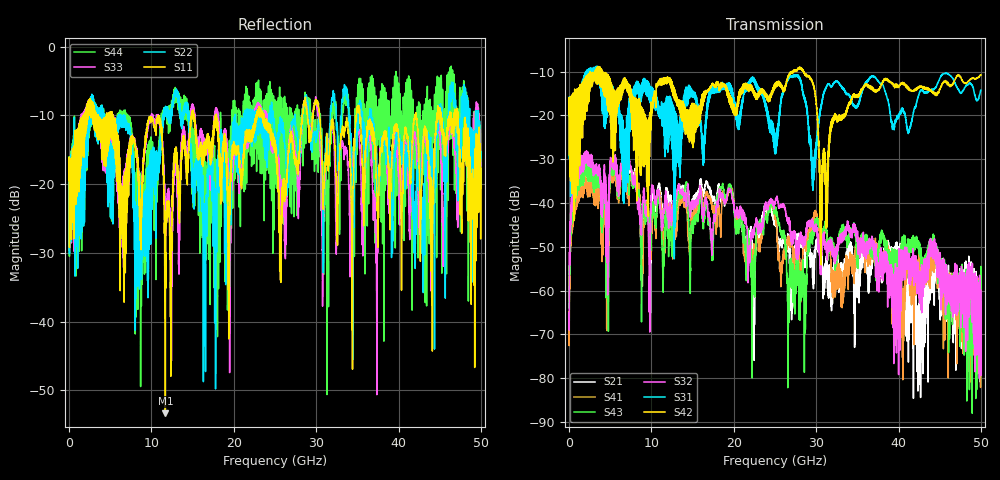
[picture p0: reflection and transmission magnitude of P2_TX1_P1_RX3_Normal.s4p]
!Keysight Technologies,N5225B,MY57041031,A.13.20.10
!Date: Friday, May 31, 2019 11:17:59
!Correction: S11(Full 4 Port(1,2,3,4))
!S12(Full 4 Port(1,2,3,4))
!S13(Full 4 Port(1,2,3,4))
!S14(Full 4 Port(1,2,3,4))
!S21(Full 4 Port(1,2,3,4))
!S22(Full 4 Port(1,2,3,4))
!S23(Full 4 Port(1,2,3,4))
!S24(Full 4 Port(1,2,3,4))
!S31(Full 4 Port(1,2,3,4))
!S32(Full 4 Port(1,2,3,4))
!S33(Full 4 Port(1,2,3,4))
!S34(Full 4 Port(1,2,3,4))
!S41(Full 4 Port(1,2,3,4))
!S42(Full 4 Port(1,2,3,4))
!S43(Full 4 Port(1,2,3,4))
!S44(Full 4 Port(1,2,3,4))
!S4P File: Measurements: <S11,S12,S13,S14>,
!<S21,S22,S23,S24>,
!<S31,S32,S33,S34>,
!<S41,S42,S43,S44>:
# Hz S  dB  R 50.0
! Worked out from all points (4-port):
!   5000 points, 10 MHz to 50 GHz, reference 50 ohm
!   strongest paths, dB at 10 MHz, 12.51 GHz, 25.01 GHz, 37.51 GHz, 50 GHz:
!     S42: -19.7, -14.1, -12.9, -14.2, -10.7
!     S31: -19.5, -17.3, -28.8, -12.1, -14.2
!     S32: -65.1, -42.4, -40.2, -56.7, -63.4
!     S43: -62.3, -46.9, -42.0, -50.8, -61.4
!     S41: -64.8, -44.4, -43.4, -51.4, -67.8
!     S21: -62.4, -42.2, -44.5, -52.7, -71.1
!   lowest |S11| = -53.4 dB at 11.69 GHz (marker M1), VSWR 1.00, Z = 49.8 - j0.101 ohm
!   |S11| at or under -10 dB: 5.36 GHz to 10.81 GHz (5.45 GHz wide, 67.4 % of centre); 17.89 GHz to 22.7 GHz (4.805 GHz wide, 23.7 % of centre); 35.31 GHz to 41.96 GHz (6.644 GHz wide, 17.2 % of centre)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
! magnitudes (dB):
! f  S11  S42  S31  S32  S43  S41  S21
! 10 MHz  -19.4  -19.7  -19.5  -65.1  -62.3  -64.8  -62.4
! 2.02 GHz  -11.4  -18.0  -12.1  -28.4  -30.3  -32.0  -30.0
! 11.69 GHz  -53.4  -11.6  -22.8  -38.2  -42.8  -44.0  -38.7
! 16.51 GHz  -14.0  -14.7  -26.3  -39.5  -41.6  -39.1  -36.1
! 28.17 GHz  -12.0  -9.1  -12.7  -47.5  -62.2  -57.2  -48.9
! 30.63 GHz  -13.7  -40.3  -17.9  -51.7  -46.4  -47.5  -52.1
! 50 GHz  -17.7  -10.7  -14.2  -63.4  -61.4  -67.8  -71.1
